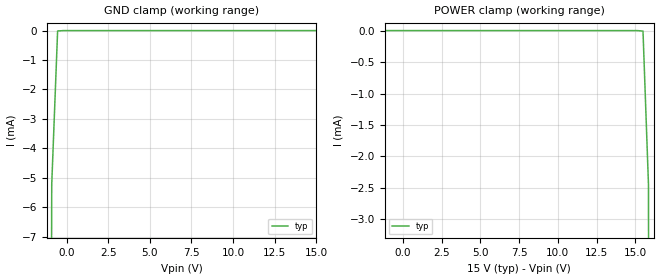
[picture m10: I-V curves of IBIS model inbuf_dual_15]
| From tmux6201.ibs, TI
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| inbuf_dual_15
[Model]   inbuf_dual_15
Model_type   Input
Vinl = 0.8
Vinh = 1.3
|   typ   min   max
C_comp   4.014581e-13   NA   NA
[Voltage Range]   15   NA   NA
[Temperature Range]   27   NA   NA
[Power Clamp Reference]   15   NA   NA
[GND Clamp Reference]   0   NA   NA
[GND Clamp]
|   Voltage   I(typ)   I(min)   I(max)
-20V      -5.936A    NA         NA
-1.263V   -72.13mA   NA         NA
-909.1mV  -5.221mA   NA         NA
-555.6mV  -13.09uA   NA         NA
15V       515nA      NA         NA
[POWER Clamp]
|   Voltage   I(typ)   I(min)   I(max)
-5V       515.1nA    NA         NA
15.51V    -7.81uA    NA         NA
15.86V    -2.444mA   NA         NA
16.21V    -58.83mA   NA         NA
30V       -4.366A    NA         NA
